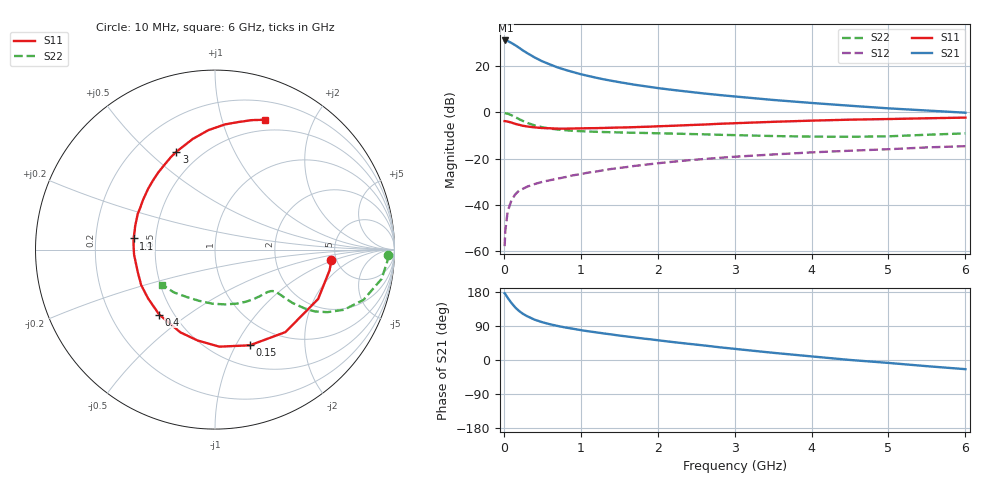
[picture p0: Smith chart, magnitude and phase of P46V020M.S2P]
! SIEMENS Small Signal Semiconductors
! BFP182
! Si NPN RF Bipolar Junction Transistor in SOT143
! VCE = 6 V  IC = 20 mA
! Common Emitter S-Parameters:  March  1996
# GHz  S  MA  R  50
!  f  S11  S21  S12  S22
! GHz  MAG  ANG  MAG  ANG  MAG  ANG  MAG  ANG
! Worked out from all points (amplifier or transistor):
!   36 points, 10 MHz to 6 GHz, reference 50 ohm
!   highest |S21| = 31.1 dB at 20 MHz (marker M1)
!   |S21| within 3 dB of that: start of sweep to 191.2 MHz
!   unconditionally stable (mu >= 1): 885.9 MHz to 5.444 GHz
!   at 250 MHz: K = 0.47, MSG = 29.8 dB, |S12| = -32.9 dB
!   at 1.4 GHz: K = 1.12, MAG = 17.0 dB, |S12| = -24.4 dB
!   at 6 GHz: K = 0.94, MSG = 7.2 dB, |S12| = -14.5 dB
!   S11 on the Smith chart (normalised r, x): 10 MHz: 4.55, -0.90; 150 MHz: 0.73, -1.14; 400 MHz: 0.42, -0.39; 1.1 GHz: 0.37, +0.06; 3 GHz: 0.37, +0.62; 6 GHz: 0.38, +1.39
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0.01  0.6515 -5.0  35.78 176.2  0.0013 84.7  0.9659 -1.7
0.02  0.6488 -10.2  35.91 173.7  0.0029 83.0  0.9624 -3.9
0.05  0.6371 -25.6  34.91 164.1  0.0073 80.8  0.9423 -10.0
0.1  0.6044 -49.5  31.6 150.2  0.0129 67.0  0.8734 -18.7
0.15  0.5675 -70.0  28.24 138.3  0.0172 61.1  0.7931 -25.0
0.2  0.5413 -87.4  24.86 129.0  0.0208 56.9  0.7168 -29.1
0.25  0.5158 -100.7  21.74 121.6  0.0226 53.5  0.6538 -31.8
0.3  0.4999 -112.7  19.31 115.9  0.0249 52.4  0.6001 -33.2
0.4  0.4771 -130.7  15.45 106.4  0.0285 50.8  0.5266 -34.5
0.5  0.4614 -144.0  12.73 99.7  0.0318 49.6  0.4801 -34.7
0.6  0.4563 -154.3  10.9 94.3  0.0345 51.0  0.4494 -34.6
0.7  0.4484 -163.2  9.377 89.8  0.0373 51.6  0.4286 -34.7
0.9  0.4518 -176.4  7.46 82.4  0.044 52.3  0.4025 -35.2
1.1  0.4578 172.2  6.142 75.7  0.0505 52.5  0.3879 -36.6
1.5  0.4741 155.4  4.519 64.5  0.0635 52.2  0.3714 -40.7
1.8  0.4894 144.3  3.765 56.9  0.0732 50.8  0.3621 -45.0
2.2  0.517 132.1  3.066 47.3  0.0865 48.2  0.3506 -51.6
3  0.5863 111.5  2.219 29.4  0.1109 41.6  0.3247 -68.0
3.5  0.6288 101.4  1.866 19.0  0.1241 37.1  0.3101 -79.9
4.5  0.7 85.4  1.399 0.1  0.1495 28.5  0.2987 -107.0
5.5  0.7501 74.1  1.103 -16.3  0.1764 20.7  0.3308 -133.9
6  0.7753 68.9  0.989 -24.2  0.1873 15.8  0.354 -146.6
